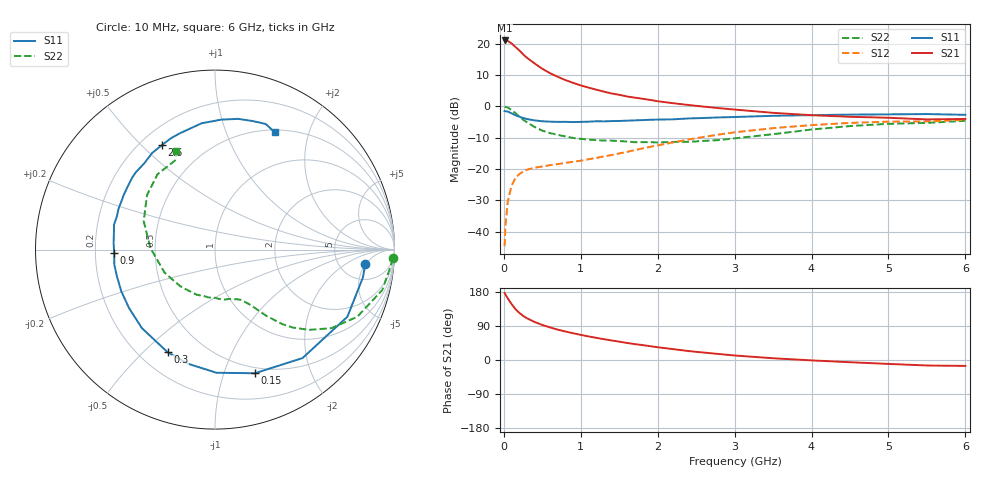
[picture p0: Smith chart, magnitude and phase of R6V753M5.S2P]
! SIEMENS Small Signal Semiconductors
! BFR193
! Si NPN RF Bipolar Junction Transistor in SOT23
! VCE = 0.75 V  IC = 3.5 mA
! Common Emitter S-Parameters:  May  1996
# GHz  S  MA  R  50
!  f  S11  S21  S12  S22
! GHz  MAG  ANG  MAG  ANG  MAG  ANG  MAG  ANG
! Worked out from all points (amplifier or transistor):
!   36 points, 10 MHz to 6 GHz, reference 50 ohm
!   highest |S21| = 21.0 dB at 10 MHz (marker M1)
!   |S21| within 3 dB of that: start of sweep to 192.9 MHz
!   unconditionally stable (mu >= 1): 955.8 MHz to 2.28 GHz; 5.781 GHz to end of sweep
!   at 250 MHz: K = 0.34, MSG = 18.7 dB, |S12| = -20.8 dB
!   at 1.4 GHz: K = 1.10, MAG = 7.9 dB, |S12| = -15.5 dB
!   at 6 GHz: K = 1.00, MAG = -0.1 dB, |S12| = -4.3 dB
!   S11 on the Smith chart (normalised r, x): 10 MHz: 9, -5; 150 MHz: 0.44, -1.28; 300 MHz: 0.31, -0.59; 900 MHz: 0.28, -0.02; 2.6 GHz: 0.28, +0.58; 6 GHz: 0.53, +1.50
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0.01  0.8413 -5.4  11.27 176.8  0.0059 86.7  0.9919 -2.8
0.02  0.8386 -10.7  11.13 173.0  0.012 83.6  0.983 -5.4
0.05  0.827 -26.9  11.08 162.9  0.0297 76.1  0.9588 -13.6
0.1  0.7765 -51.1  10.11 147.8  0.0542 64.3  0.8763 -25.3
0.15  0.7239 -72.1  8.893 134.5  0.072 55.6  0.7828 -34.0
0.2  0.6863 -89.3  7.832 124.6  0.083 49.0  0.6898 -40.4
0.25  0.6535 -103.2  6.774 116.6  0.0913 44.3  0.6146 -45.0
0.3  0.6296 -114.8  5.973 110.2  0.0977 41.6  0.5593 -47.9
0.4  0.5978 -132.9  4.841 100.3  0.1052 38.2  0.4694 -52.1
0.5  0.5793 -145.8  3.979 92.5  0.1102 37.1  0.4106 -54.8
0.6  0.5713 -156.1  3.39 86.0  0.1156 37.1  0.3758 -56.7
0.7  0.5663 -164.5  2.966 80.1  0.1201 37.9  0.3518 -58.6
0.9  0.5623 -177.9  2.375 70.6  0.1309 41.1  0.314 -63.1
1.1  0.5706 170.8  1.996 62.3  0.1436 44.3  0.2963 -68.7
1.3  0.5771 161.5  1.721 54.9  0.1592 47.1  0.2854 -74.5
1.6  0.5924 149.3  1.441 45.0  0.1882 50.3  0.2759 -85.4
2.2  0.6218 129.3  1.125 28.7  0.2667 50.3  0.2714 -112.2
2.6  0.6532 116.8  0.991 19.6  0.3262 46.7  0.2814 -133.8
3.5  0.7079 96.0  0.79 4.6  0.4501 32.6  0.3602 178.5
4.5  0.7398 79.9  0.683 -5.9  0.5454 15.6  0.4856 141.2
5.5  0.7549 68.1  0.62 -14.5  0.5764 -0.3  0.546 113.4
6  0.734 62.9  0.631 -15.6  0.6083 -4.9  0.5896 111.4
